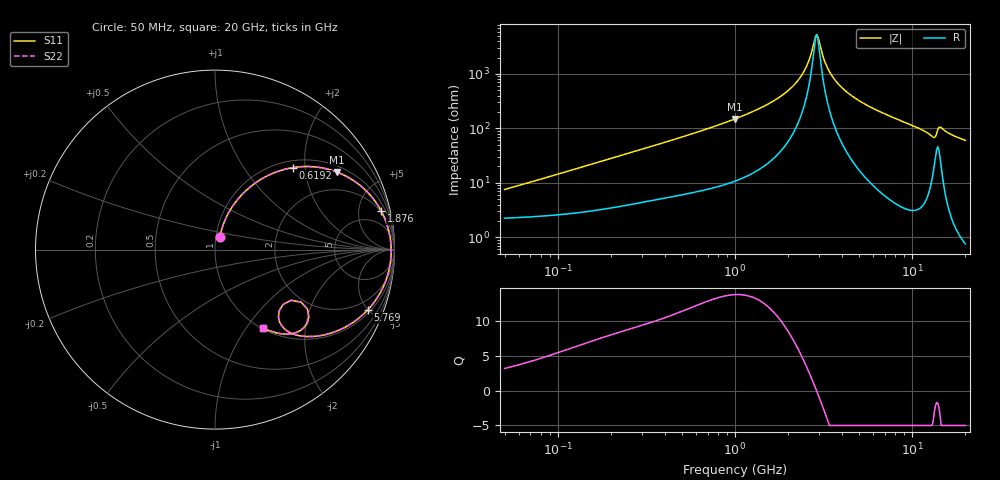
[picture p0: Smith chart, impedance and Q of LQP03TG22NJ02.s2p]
!Murata Part Number: LQP03TG22NJ02
!These Parameters are Measured in Series Mode Connection
!  o--[Z]--o
!Port1  Port2
!  o-------o
!Freq. Start=50[MHz] Stop=20[GHz], 401[Steps]
# Hz S RI R 50
!Freq.(Hz) S11(Real) S11(Imag) S21(Real) S21(Imag) S12(Real) S12(Imag) S22(Real) S22(Imag)
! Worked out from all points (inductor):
!   401 points, 50 MHz to 20 GHz, reference 50 ohm
!   read as one part in series: L = 22.9 nH near 51.52 MHz
!   highest Q = 13.9 at 1 GHz (marker M1), where L = 23.7 nH
!   self-resonance near 2.853 GHz
!   S11 on the Smith chart (normalised r, x): 50 MHz: 1.04, +0.14; 619.2 MHz: 1.14, +1.72; 1.876 GHz: 1.87, +8.39; 5.769 GHz: 1.21, -4.99; 20 GHz: 1.02, -1.21
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5e7  0.0268 0.0689  0.9732 -0.0689  0.9732 -0.0689  0.0268 0.0689
1.364002e8  0.061 0.176  0.939 -0.176  0.939 -0.176  0.061 0.176
3.721004e8  0.2311 0.3755  0.7689 -0.3755  0.7689 -0.3755  0.2311 0.3755
6.192061e8  0.4332 0.4568  0.5668 -0.4568  0.5668 -0.4568  0.4332 0.4568
1e9  0.6788 0.4323  0.3212 -0.4323  0.3212 -0.4323  0.6788 0.4323
1.432596e9  0.8419 0.3277  0.1581 -0.3277  0.1581 -0.3277  0.8419 0.3277
1.875929e9  0.9269 0.2134  0.0731 -0.2134  0.0731 -0.2134  0.9269 0.2134
2.383959e9  0.9698 0.0976  0.0302 -0.0976  0.0302 -0.0976  0.9698 0.0976
2.569357e9  0.9768 0.0599  0.0232 -0.0599  0.0232 -0.0599  0.9768 0.0599
2.728004e9  0.9801 0.0295  0.0199 -0.0295  0.0199 -0.0295  0.9801 0.0295
2.896447e9  0.9815 -0.00106  0.0185 0.00106  0.0185 0.00106  0.9815 -0.00106
3.265178e9  0.9784 -0.0624  0.0216 0.0624  0.0216 0.0624  0.9784 -0.0624
3.680849e9  0.9672 -0.1234  0.0328 0.1234  0.0328 0.1234  0.9672 -0.1234
4.405649e9  0.9352 -0.2126  0.0648 0.2126  0.0648 0.2126  0.9352 -0.2126
5.769027e9  0.852 -0.3351  0.148 0.3351  0.148 0.3351  0.852 -0.3351
7.442007e9  0.7359 -0.4265  0.2641 0.4265  0.2641 0.4265  0.7359 -0.4265
1.149051e10  0.4638 -0.4784  0.5362 0.4784  0.5362 0.4784  0.4638 -0.4784
1.295331e10  0.361 -0.4053  0.639 0.4053  0.639 0.4053  0.361 -0.4053
1.375312e10  0.4252 -0.2825  0.5748 0.2825  0.5748 0.2825  0.4252 -0.2825
1.438523e10  0.5229 -0.3769  0.4771 0.3769  0.4771 0.3769  0.5229 -0.3769
1.550395e10  0.4402 -0.4658  0.5598 0.4658  0.5598 0.4658  0.4402 -0.4658
2e10  0.2693 -0.4374  0.7307 0.4374  0.7307 0.4374  0.2693 -0.4374
